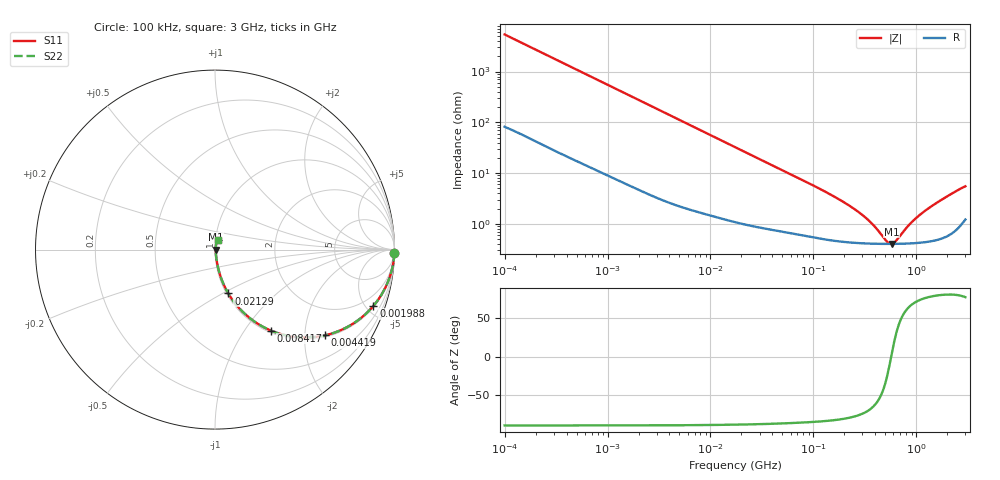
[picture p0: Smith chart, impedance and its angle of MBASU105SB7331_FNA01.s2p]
! MBASU105SB7331_FNA01  S-PARAMETER MODEL  ( Standard Model )
! Model Generated by TAIYO YUDEN Corporation (http://www.ty-top.com)
! Version 1.0
! TAIYO YUDEN Control No. 220601
! Copyright(c) 2017 TAIYO YUDEN CO.,LTD. All Rights Reserved.
! Product Description (link to TY-COMPAS)
! https://ds.yuden.co.jp/TYCOMPAS/or/detail?pn=MBASU105SB7331KFNA01&u=M
! Products Name : Multilayer Ceramic Capacitors
! Characteristics :
!  Capacitance : 330 [pF] , Rated Voltage : 50 [V] , TCC : X7R
!  Case Size : 1.0 x 0.5 / 0.039 x 0.02 [mm/inch] , Thickness : 0.5 / 0.02 [mm/inch]
!  (Conditions: Temperature = 25 [degC] , DC Bias Voltage = 0 [V])
! External Node Assignments :
!  1  o---| |---o  2
! GND o---------o GND
! Frequency Range : 100kHz  -  3GHz  [ 401 STEP ]
# MHZ S RI R 50
! Freq[MHz].  S11 Real  S11 Imag  S21 Real  S21 Imag  S12 Real  S12 Imag  S22 Real  S22 Imag
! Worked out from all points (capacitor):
!   401 points, 100 kHz to 3 GHz, reference 50 ohm
!   read as one part in series: C = 295 pF near 105.3 kHz
!   lowest |Z| = 404 mohm at 576.5 MHz (marker M1)
!   series resonance near 570.1 MHz, so ESL is about 260 pH
!   S11 on the Smith chart (normalised r, x): 100 kHz: open; 1.988 MHz: 1.09, -5.58; 4.419 MHz: 1.05, -2.53; 8.417 MHz: 1.03, -1.34; 21.29 MHz: 1.02, -0.53; 3 GHz: 1.02, +0.11
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0.1  0.9994 -0.0186  0.000627 0.0186  0.000627 0.0186  0.9994 -0.0186
0.562235  0.988 -0.1012  0.012 0.1012  0.012 0.1012  0.988 -0.1012
1.156955  0.9549 -0.1994  0.0451 0.1994  0.0451 0.1994  0.9549 -0.1994
1.987766  0.8822 -0.3141  0.1178 0.3141  0.1178 0.3141  0.8822 -0.3141
3.161081  0.7527 -0.4227  0.2473 0.4227  0.2473 0.4227  0.7527 -0.4227
4.419184  0.6131 -0.4776  0.3869 0.4776  0.3869 0.4776  0.6131 -0.4776
8.417093  0.3126 -0.4517  0.6874 0.4517  0.6874 0.4517  0.3126 -0.4517
12.07428  0.1861 -0.3754  0.8139 0.3754  0.8139 0.3754  0.1861 -0.3754
17.7727  0.1001 -0.2839  0.8999 0.2839  0.8999 0.2839  0.1001 -0.2839
21.28644  0.0743 -0.2445  0.9257 0.2445  0.9257 0.2445  0.0743 -0.2445
42.68829  0.0246 -0.1296  0.9754 0.1296  0.9754 0.1296  0.0246 -0.1296
97.38194  0.00879 -0.0576  0.9912 0.0576  0.9912 0.0576  0.00879 -0.0576
180.7614  0.00535 -0.0292  0.9947 0.0292  0.9947 0.0292  0.00535 -0.0292
280.1453  0.00442 -0.016  0.9956 0.016  0.9956 0.016  0.00442 -0.016
371.9668  0.00415 -0.00913  0.9959 0.00913  0.9959 0.00913  0.00415 -0.00913
547.5153  0.00402 -0.00084  0.996 0.00084  0.996 0.00084  0.00402 -0.00084
576.4768  0.00402 0.000232  0.996 -0.000232  0.996 -0.000232  0.00402 0.000232
622.8167  0.00403 0.00184  0.996 -0.00184  0.996 -0.00184  0.00403 0.00184
870.6963  0.00419 0.0091  0.9958 -0.0091  0.9958 -0.0091  0.00419 0.0091
1156.079  0.00455 0.0161  0.9954 -0.0161  0.9954 -0.0161  0.00455 0.0161
1886.474  0.00641 0.0318  0.9936 -0.0318  0.9936 -0.0318  0.00641 0.0318
3000  0.0148 0.0523  0.9852 -0.0523  0.9852 -0.0523  0.0148 0.0523
